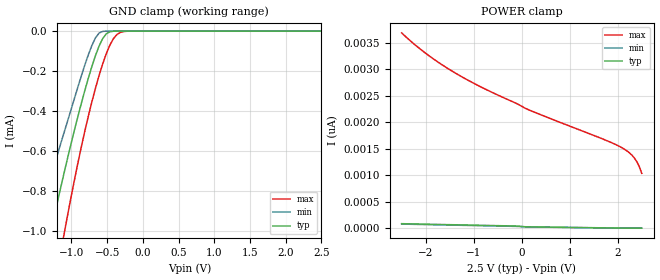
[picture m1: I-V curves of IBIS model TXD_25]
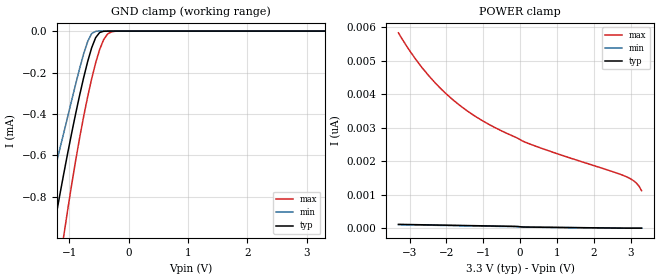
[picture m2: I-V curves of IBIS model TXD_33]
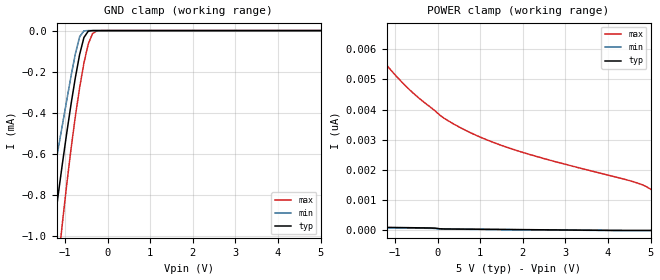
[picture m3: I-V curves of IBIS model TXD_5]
| IBIS file created by Layout Workbench Version 22.1.4.12161.401368   004
| Cadence Design Systems, Inc. 2011
[IBIS ver]   4.2
[File name]  iso6463.ibs
[File Rev]   1.5
[Date]   05 15, 2025
[Source]   Model built from TISPICED simulations at:
   Texas Instruments Incorporated.
   Analog-eLab, HPA 12500 TI Blvd
   Dallas, TX -75243
   For Support e-mail: elab_ibis@list.ti.com
[Notes]   This product is designed as an aid for customers of Texas Instruments.
   No warranties, either expressed or implied, with respect to this third party software (if any)
   or with respect to its fitness for any particular purpose is claimed by Texas Instruments or
   the author. The software (if any) is provided solely on an "as is" basis. The entire risk as to
   its quality and performance is with the customer
[Disclaimer] This product is designed as an aid for customers of Texas Instruments. No warranties, either expressed or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
[Copyright] (C)Copyright 2025 Texas Instruments Incorporated. All rights reserved.
|   ISO6463DW
[Component] ISO6463DW
[Manufacturer] Texas Instruments Incorporated
[Package]   |16-pin SOIC DW package
|   typ   min   max
R_pkg   0.13983   0.12494   0.17928
L_pkg   2.1802nH   1.92454nH   2.85707nH
C_pkg   0.42060pF   0.21450pF   0.61276pF
[Pin]  signal_name   model_name   R_pin   L_pin   C_pin
1   VCC1   POWER   0.09703   2.25823nH  0.63889pF
2   INA   TXD1   0.10567   2.15194nH  0.30706pF
3   INB   TXD1   0.12889   1.99554nH  0.21450pF
4   INC   TXD1   0.12623   1.94755nH  0.61276pF
5   OUTD   RXD1   0.12494   1.92646nH  0.36666pF
6   OUTE   RXD1   0.12883   1.99615nH  0.50841pF
7   OUTF   RXD1   0.17807   2.83638nH  0.45904pF
8   GND1   GND   0.08216   2.43955nH  0.44498pF
9   GND2   GND   0.10126   2.44074nH  0.40934pF
10   INF   TXD1   0.17928   2.85707nH  0.52717pF
11   INE   TXD1   0.14038   2.18765nH  0.43235pF
12   IND   TXD1   0.12617   1.94399nH  0.32633pF
13   OUTC   RXD1   0.12498   1.92454nH  0.37783pF
14   OUTB   RXD1   0.14050   2.18615nH  0.38097pF
15   OUTA   RXD1   0.08275   2.09014nH  0.75096pF
16   VCC2   POWER   0.09747   2.26909nH  0.67439pF
|   ISO6463FDW
[Component]   ISO6463FDW
[Manufacturer]   TI
[Package]   |16 SOIC - DW package
|   typ   min   max
R_pkg   0.13983   0.12494   0.17928
L_pkg   2.1802nH   1.92454nH   2.85707nH
C_pkg   0.42060pF   0.21450pF   0.61276pF
[Pin]  signal_name   model_name   R_pin   L_pin   C_pin
1   VCC1   POWER   0.09703   2.25823nH  0.63889pF
2   INA   TXD2   0.10567   2.15194nH  0.30706pF
3   INB   TXD2   0.12889   1.99554nH  0.21450pF
4   INC   TXD2   0.12623   1.94755nH  0.61276pF
5   OUTD   RXD1   0.12494   1.92646nH  0.36666pF
6   OUTE   RXD1   0.12883   1.99615nH  0.50841pF
7   OUTF   RXD1   0.17807   2.83638nH  0.45904pF
8   GND1   GND   0.08216   2.43955nH  0.44498pF
9   GND2   GND   0.10126   2.44074nH  0.40934pF
10   INF   TXD2   0.17928   2.85707nH  0.52717pF
11   INE   TXD2   0.14038   2.18765nH  0.43235pF
12   IND   TXD2   0.12617   1.94399nH  0.32633pF
13   OUTC   RXD1   0.12498   1.92454nH  0.37783pF
14   OUTB   RXD1   0.14050   2.18615nH  0.38097pF
15   OUTA   RXD1   0.08275   2.09014nH  0.75096pF
16   VCC2   POWER   0.09747   2.26909nH  0.67439pF
|   Model Selectors
[Model Selector] TXD1
TXD_25   TXD Input model for 2.25V - 2.75V
TXD_33   TXD Input model for 3.0V - 3.6V
TXD_5   TXD Input model for 4.5V - 5.5V
[Model Selector] RXD1
RXD_25   RXD Output model for 2.25V - 2.75V
RXD_33   RXD Output model for 3.0V - 3.6V
RXD_5   RXD Output model for 4.5V - 5.5V
[Model Selector] EN
EN_25   TXD Input model for 2.25V - 2.75V
EN_33   TXD Input model for 3.15V - 3.6V
EN_5   TXD Input model for 4.5V - 5.5V
[Model Selector] TXD2
TXDF_25   TXD Input model for 2.25V - 2.75V
TXDF_33   TXD Input model for 3.0V - 3.6V
TXDF_5   TXD Input model for 4.5V - 5.5V
| Models and submodels in the file (12): TXD_25 (Input), TXD_33 (Input), TXD_5 (Input), TXDF_25 (Input), TXDF_33 (Input), TXDF_5 (Input), EN_25 (Input), EN_33 (Input), EN_5 (Input), RXD_25 (3-state), RXD_33 (3-state), RXD_5 (3-state)
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|   TXD_25 Model
[Model]   TXD_25
Model_type   Input
|Signals   TXD
Vinl =  0.750V
Vinh =  1.750V
|   typ   min   max
C_comp   1.3pF   1.1pF   1.5pF
|   typ   min   max
[Temperature Range]   27   -40   125
[Voltage range]   2.5V   2.25V   2.75V
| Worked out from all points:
|   GND clamp passes 1 mA (typ) near -1.29 V on its own axis
[GND_clamp]
|Voltage   I(typ)   I(min)   I(max)
-2.5V     -3.261mA   -2.697mA   -4.025mA
-1.48V    -1.333mA   -1.01mA    -1.787mA
-1.276V   -983uA     -716.4uA   -1.36mA
-1.123V   -739.3uA   -529.9uA   -1.053mA
-1.072V   -661.5uA   -470.4uA   -954.6uA
-919mV    -439.5uA   -290uA     -675.2uA
-766mV    -238.2uA   -120.7uA   -428.7uA
-613mV    -74.62uA   -9.78uA    -221.8uA
-511mV    -13.26uA   -161.8nA   -111.7uA
-409mV    -630.3nA   -1.04nA    -36.14uA
-256mV    -2.009nA   -6.036pA   -1.659uA
2.5V      0A         0A         0A
[POWER_clamp]
|Voltage   I(typ)   I(min)   I(max)
-2.5V     84.61pA    76.91pA    3.684nA
-2.192V   78.79pA    71.19pA    3.438nA
-1.835V   72.09pA    64.59pA    3.191nA
-1.427V   64.46pA    57.09pA    2.951nA
-1.019V   56.88pA    49.63pA    2.744nA
154mV     24.79pA    22.52pA    2.229nA
1.684V    6.302pA    4.156pA    1.684nA
2.092V    1.394pA    0A         1.515nA
2.245V    0A         0A         1.42nA
2.347V    0A         0A         1.323nA
2.449V    0A         0A         1.162nA
2.5V      0A         0A         1.034nA
|   TXD_33 Model
[Model]   TXD_33
Model_type   Input
|Signals   TXD
Vinl =  0.990V
Vinh =  2.310V
|   typ   min   max
C_comp   1.3pF   1.1pF   1.5pF
|   typ   min   max
[Temperature Range]   27   -40   125
[Voltage range]   3.3V   3.0V   3.6V
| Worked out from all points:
|   GND clamp passes 1 mA (typ) near -1.29 V on its own axis
[GND_clamp]
|Voltage   I(typ)   I(min)   I(max)
-3.3V     -4.822mA   -4.059mA   -5.82mA
-1.491V   -1.352mA   -1.027mA   -1.81mA
-1.424V   -1.234mA   -925uA     -1.668mA
-1.29V    -1.006mA   -734.8uA   -1.389mA
-1.223V   -896.7uA   -649.1uA   -1.252mA
-1.089V   -687.3uA   -490.2uA   -987.2uA
-754mV    -223.6uA   -108.8uA   -410.9uA
-620mV    -80.65uA   -12.05uA   -230.3uA
-553mV    -31.67uA   -1.049uA   -153.7uA
-419mV    -886.2nA   -1.734nA   -41.6uA
-218mV    -449.6pA   -6.494pA   -628.3nA
3.3V      0A         0A         0A
[POWER_clamp]
|Voltage   I(typ)   I(min)   I(max)
-3.3V     113.7pA    104.6pA    5.836nA
-3.065V   109.2pA    100.1pA    5.419nA
-2.797V   104pA      95.04pA    4.996nA
-2.328V   94.97pA    86.22pA    4.372nA
-1.792V   84.76pA    76.21pA    3.81nA
-1.256V   74.65pA    66.26pA    3.373nA
-720mV    64.61pA    56.39pA    3.029nA
151mV     33.16pA    30.36pA    2.565nA
2.898V    0A         0A         1.532nA
3.166V    0A         0A         1.339nA
3.233V    0A         0A         1.249nA
3.3V      0A         0A         1.12nA
|   TXD_5 Model
[Model]   TXD_5
Model_type   Input
|Signals   TXD
Vinl =  1.500V
Vinh =  3.500V
|   typ   min   max
C_comp   1.3pF   1.1pF   1.5pF
|   typ   min   max
[Temperature Range]   27   -40   125
[Voltage range]   5.0V   4.5V   5.5V
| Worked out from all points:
|   GND clamp passes 1 mA (typ) near -1.29 V on its own axis
[GND_clamp]
|Voltage   I(typ)   I(min)   I(max)
-5V       -8.158mA   -6.968mA   -9.644mA
-1.465V   -1.306mA   -987uA     -1.755mA
-1.263V   -961.6uA   -699.5uA   -1.333mA
-1.162V   -799.9uA   -575.6uA   -1.13mA
-1.061V   -645uA     -457.5uA   -933.6uA
-758mV    -228.5uA   -112.7uA   -416.8uA
-657mV    -115.6uA   -29.62uA   -276.8uA
-556mV    -33.38uA   -1.189uA   -156.8uA
-455mV    -2.832uA   -10.7nA    -64.96uA
-354mV    -87.76nA   -69.95pA   -14.52uA
-253mV    -1.79nA    -9.666pA   -1.545uA
5V        0A         0A         0A
[POWER_clamp]
|Voltage   I(typ)   I(min)   I(max)
-5V       179.5pA    164pA      20.45nA
-1.868V   115.6pA    102.9pA    6.803nA
-1.767V   113.6pA    101pA      6.576nA
-1.262V   103.8pA    91.4pA     5.583nA
-757mV    94.06pA    81.91pA    4.792nA
51mV      56.19pA    49.29pA    3.815nA
455mV     46.94pA    42.18pA    3.461nA
1.061V    39.62pA    34.91pA    3.053nA
1.768V    31.11pA    26.43pA    2.686nA
2.677V    20.17pA    15.53pA    2.309nA
4.596V    0A         0A         1.612nA
5V        0A         0A         1.364nA
